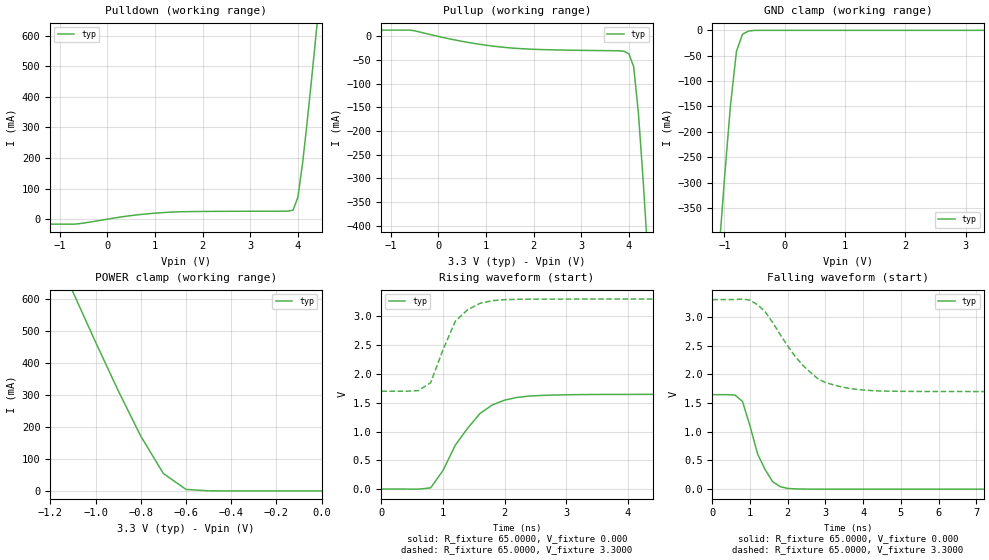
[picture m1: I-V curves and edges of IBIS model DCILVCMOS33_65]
| / 7\'7
| \ \   Xilinx Inc.
| / /
| \_\/.\   IBIS Model for Virtex-II
[IBIS ver]   2.1
[File name]   dci3365.ibs
[File Rev]   1.1
[Date]   Aug. 02, 2001
[Source]   Hspice simulations (08-02: TT, SS, FF)
[Notes]   Xilinx IBIS model for LVDCI 3.3V 65 ohms driver
[Disclaimer] The data in this model is derived from SPICE simulations using
   modeling information extracted from the target process. While
   a great deal of care has been taken to provide information
   that is accurate, this model is considered preliminary as it
   has not been verified by actual silicon measurement. Treat the
   data in this model as preliminary until actual silicon
   verification is performed.
[Copyright]   Copyright 2001, Xilinx Inc., All rights reserved
|   Component Virtex_II
[Component]   Virtex_II
[Manufacturer]   Xilinx Inc.
[Package]
| variable   typ   min   max
R_pkg   0.1000   NA   NA
L_pkg   0.8000nH   NA   NA
C_pkg   0.5000pF   NA   NA
[Pin]  signal_name   model_name   R_pin   L_pin   C_pin
io   DCILVCMOS33_65   DCILVCMOS33_65
| ins  insig   inp
| ens  ensig   inp
PGND   GND   GND
VCCO   VCCO   POWER
| Models and submodels in the file (1): DCILVCMOS33_65 (I/O)
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|   Model DCILVCMOS33_65
[Model]   DCILVCMOS33_65
Model_type   I/O
Polarity   Non-Inverting
Enable   Active-Low
Vinh = 2.0V
Vinl = 0.8V
Vmeas =   1.4000V
Cref =  35.0000pF
Rref =   1.0000M
Vref =  0.000V
C_comp   7.0000pF   NA   NA
[Temperature Range]   25.0000   NA   NA
[Voltage Range]   3.3000V   NA   NA
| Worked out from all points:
|   slope of the pulldown table from 0 to 0.495 V, typ, clamps not added: 42.9 ohm
|   slope of the pullup table from 0 to 0.495 V, typ, clamps not added: 48.1 ohm
|   GND clamp passes 1 mA (typ) near -0.57 V on its own axis
|   POWER clamp passes 1 mA (typ) near -0.52 V on its own axis
|   rising waveform, R_fixture 65.0000, V_fixture 0.000: 20-80 % time 601ps typ, NA min, NA max; typ from 0 V to 1.65 V
|   rising waveform, R_fixture 65.0000, V_fixture 3.3000: 20-80 % time 404ps typ, NA min, NA max; typ from 1.7 V to 3.3 V
|   falling waveform, R_fixture 65.0000, V_fixture 0.000: 20-80 % time 514ps typ, NA min, NA max; typ from 1.65 V to 0 V
|   falling waveform, R_fixture 65.0000, V_fixture 3.3000: 20-80 % time 1.11ns typ, NA min, NA max; typ from 3.3 V to 1.7 V
[Pulldown]
| voltage   I(typ)   I(min)   I(max)
-3.3V     -16.31mA   NA         NA
-700mV    -16.31mA   NA         NA
500mV     11.65mA    NA         NA
1.2V      21.67mA    NA         NA
3.8V      26.28mA    NA         NA
3.9V      29.65mA    NA         NA
4V        71.39mA    NA         NA
4.1V      183.8mA    NA         NA
4.2V      324.4mA    NA         NA
4.3V      475.2mA    NA         NA
4.5V      789.9mA    NA         NA
6.6V      4.263A     NA         NA
[Pullup]
| voltage   I(typ)   I(min)   I(max)
-3.3V     13.45mA    NA         NA
-600mV    13.45mA    NA         NA
500mV     -10.39mA   NA         NA
1.4V      -23.22mA   NA         NA
2.1V      -27.49mA   NA         NA
3.9V      -31.44mA   NA         NA
4V        -36.8mA    NA         NA
4.1V      -63.72mA   NA         NA
4.2V      -162.7mA   NA         NA
4.3V      -305.3mA   NA         NA
4.5V      -627.3mA   NA         NA
6.6V      -4.31A     NA         NA
[GND_clamp]
| voltage   I(typ)   I(min)   I(max)
-3.3V     -4.301A    NA         NA
-1.1V     -452.1mA   NA         NA
-1V       -293.4mA   NA         NA
-900mV    -148.1mA   NA         NA
-800mV    -41.07mA   NA         NA
-700mV    -7.668mA   NA         NA
-600mV    -1.449mA   NA         NA
-400mV    -8.141uA   NA         NA
3.3V      540.8nA    NA         NA
[POWER_clamp]
| voltage   I(typ)   I(min)   I(max)
-3.3V     4.254A     NA         NA
-1.1V     621.4mA    NA         NA
-1V       465.1mA    NA         NA
-900mV    313.6mA    NA         NA
-800mV    171.2mA    NA         NA
-700mV    54.37mA    NA         NA
-600mV    4.797mA    NA         NA
-500mV    289.2uA    NA         NA
0V        540.8nA    NA         NA
[Ramp]
| variable   typ   min   max
dV/dt_r   0.9870/0.5441n   NA   NA
dV/dt_f   0.9606/1.1061n   NA   NA
R_load = 65.0000
[Rising Waveform]
R_fixture = 65.0000
V_fixture = 0.000
| time   V(typ)   V(min)   V(max)
0s        17.08uV    NA         NA
800ps     21.59mV    NA         NA
1ns       323.1mV    NA         NA
1.2ns     763.9mV    NA         NA
1.4ns     1.057V     NA         NA
1.6ns     1.313V     NA         NA
1.8ns     1.462V     NA         NA
2.2ns     1.591V     NA         NA
3.4ns     1.643V     NA         NA
10ns      1.645V     NA         NA
[Rising Waveform]
R_fixture = 65.0000
V_fixture = 3.3000
V_fixture_min = 3.0000
V_fixture_max = 3.6000
| time   V(typ)   V(min)   V(max)
0s        1.699V     NA         NA
600ps     1.71V      NA         NA
800ps     1.847V     NA         NA
1ns       2.42V      NA         NA
1.2ns     2.916V     NA         NA
1.4ns     3.115V     NA         NA
1.6ns     3.226V     NA         NA
1.8ns     3.272V     NA         NA
2.4ns     3.299V     NA         NA
10ns      3.3V       NA         NA
[Falling Waveform]
R_fixture = 65.0000
V_fixture = 0.000
| time   V(typ)   V(min)   V(max)
0s        1.645V     NA         NA
600ps     1.638V     NA         NA
800ps     1.526V     NA         NA
1ns       1.097V     NA         NA
1.2ns     611.8mV    NA         NA
1.4ns     341.1mV    NA         NA
1.6ns     129.7mV    NA         NA
1.8ns     43.4mV     NA         NA
2.4ns     1.764mV    NA         NA
10ns      2.586uV    NA         NA
[Falling Waveform]
R_fixture = 65.0000
V_fixture = 3.3000
V_fixture_min = 3.0000
V_fixture_max = 3.6000
| time   V(typ)   V(min)   V(max)
0s        3.3V       NA         NA
800ps     3.309V     NA         NA
1.2ns     3.209V     NA         NA
1.4ns     3.09V      NA         NA
2ns       2.49V      NA         NA
2.4ns     2.156V     NA         NA
2.8ns     1.922V     NA         NA
3.4ns     1.782V     NA         NA
4.6ns     1.707V     NA         NA
10ns      1.699V     NA         NA
